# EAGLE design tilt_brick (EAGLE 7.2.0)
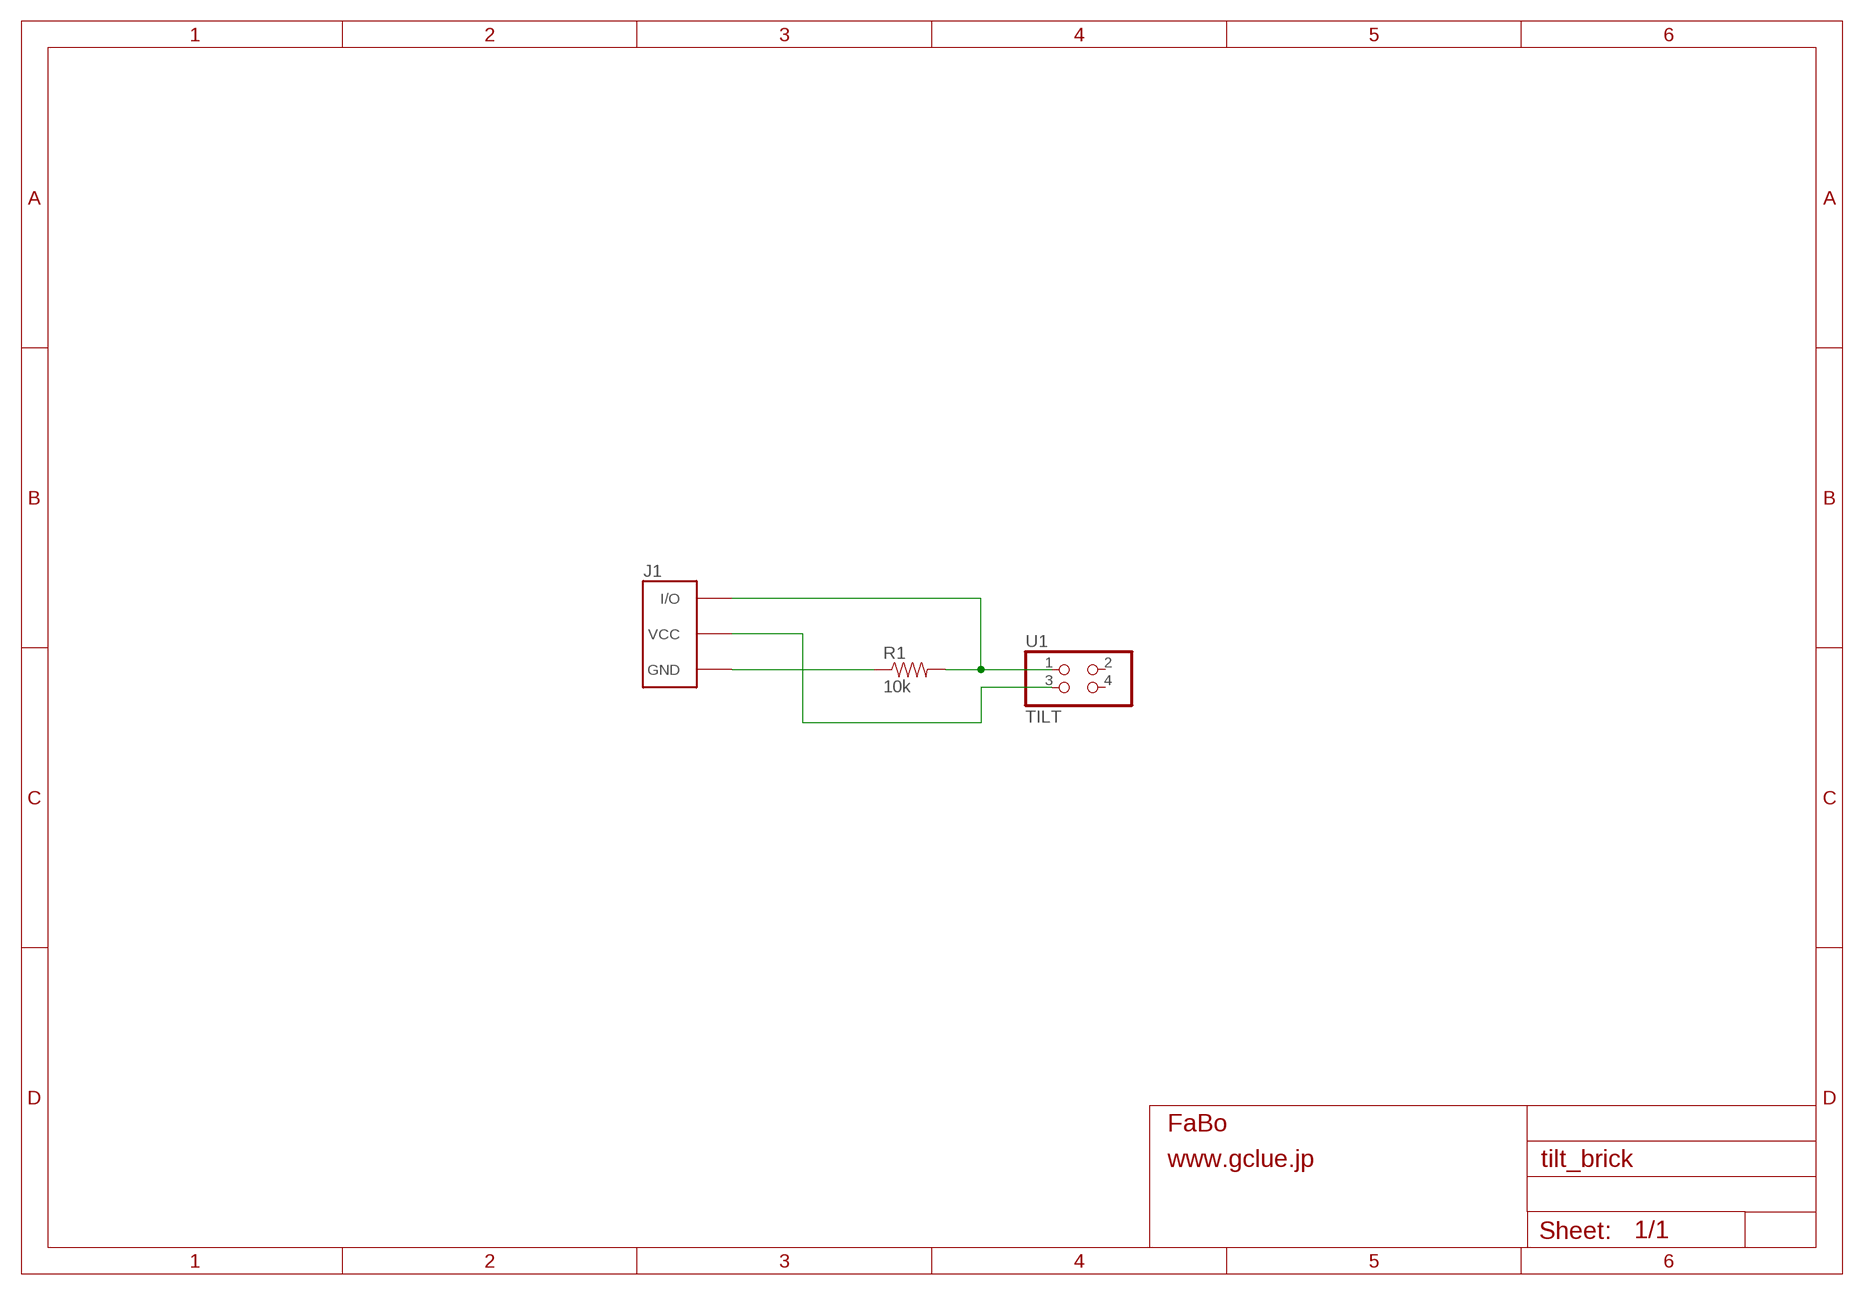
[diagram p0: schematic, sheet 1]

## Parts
J1  BRICK_3PIN  [BRICK_3PIN]
R1  10k  RESISTORKIT  [AXIAL-0.3-KIT]
U1  TILT  PINHD-2X2  [2X02]

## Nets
GND: J1.GND R1.P$1
N$3: J1.IN/OUT(I/O) R1.P$2 U1.1
N$5: J1.VCC U1.3
Unconnected: U1.2 U1.4

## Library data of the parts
J1 = Gclue:BRICK_3PIN: FaBo Brick 3pin
R1 = SparkFun:RESISTOR: Resistor
U1 = pinhead:PINHD-2X2: PIN HEADER

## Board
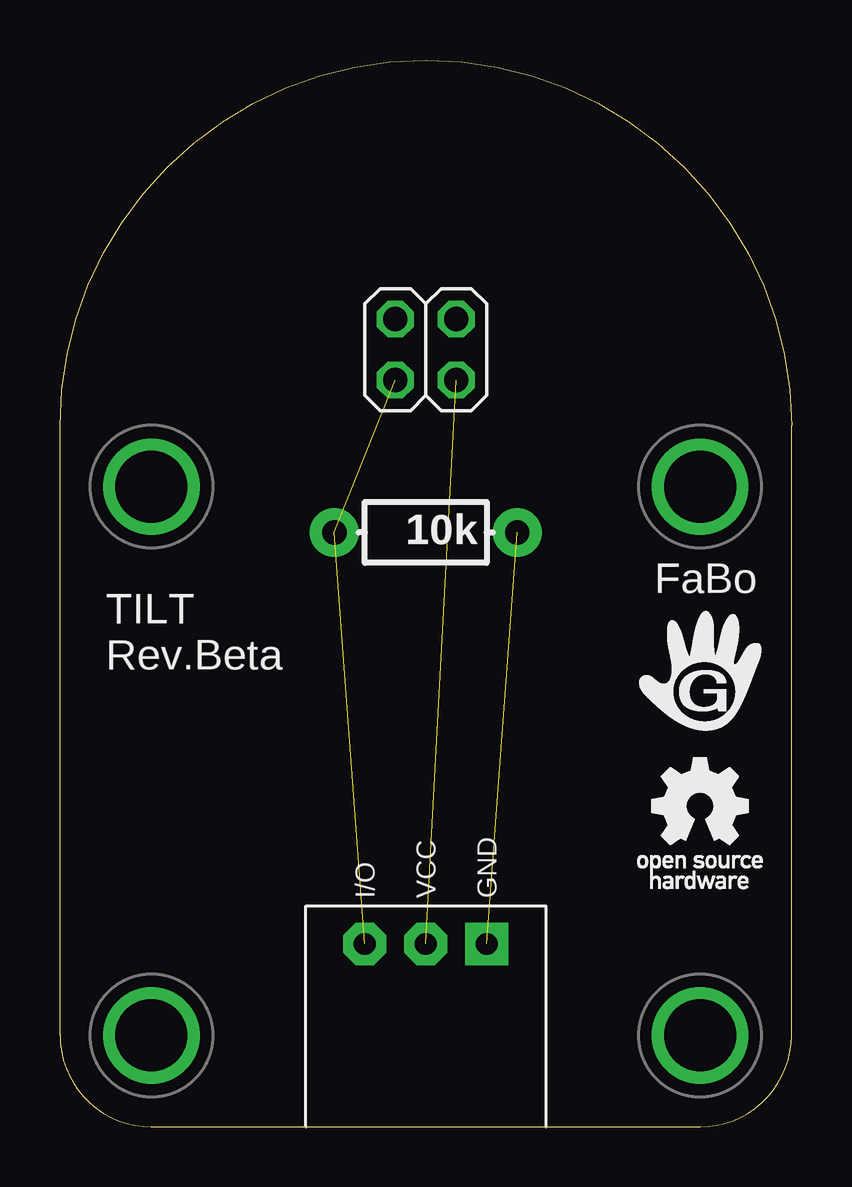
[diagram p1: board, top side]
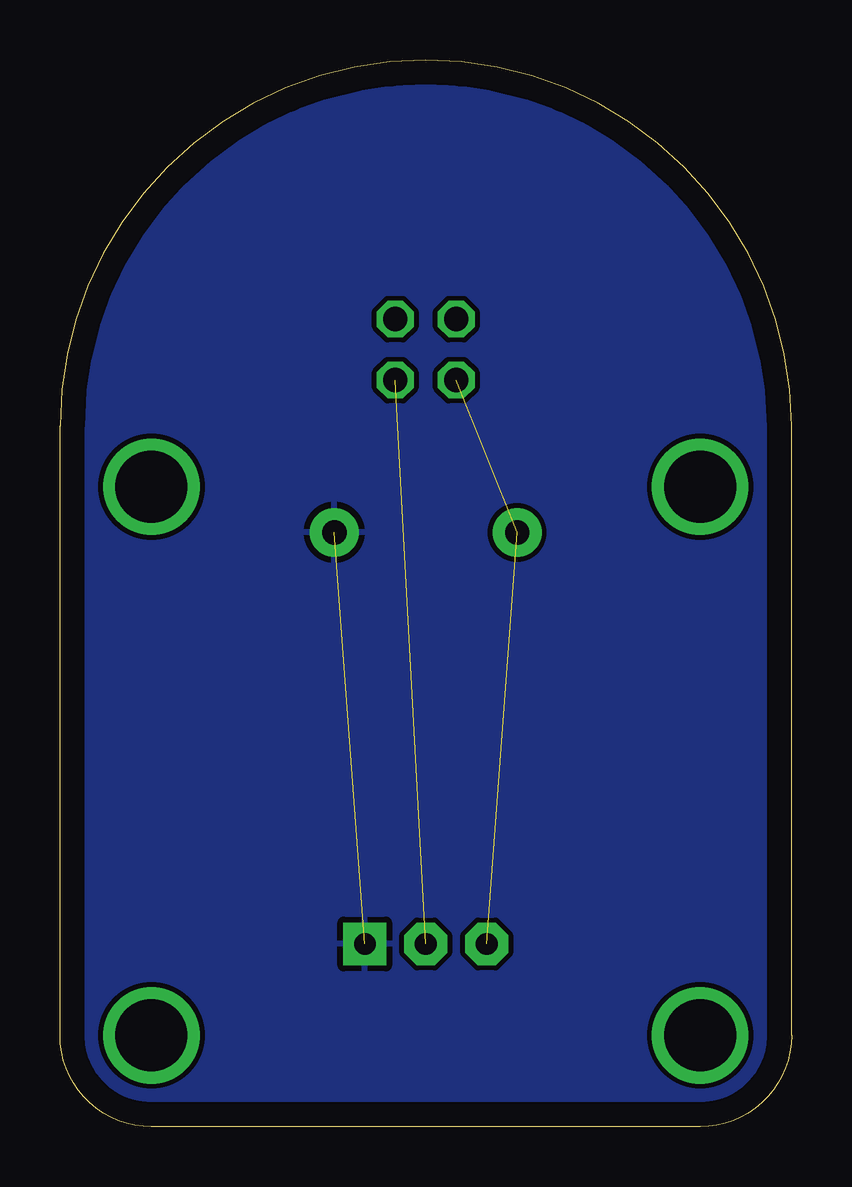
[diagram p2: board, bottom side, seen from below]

Size 30.48 x 44.45 mm. Coordinates in mm from the lower left corner, seen from the top.
Copper layers (1*16): Top 0.035mm / dielectric 1.5mm / Bottom 0.035mm
Design rules "default": minimum track width 10mil, minimum drill 24mil, track to track 8mil, track to pad 8mil, pad to pad 8mil, via to via 8mil, smd to smd 8mil, copper to edge 40mil, drill to drill 8mil, minimum pad ring 10mil, minimum via ring 8mil, stop-mask expansion 4mil, vias tented up to drill 0mil, thermal gap 10mil

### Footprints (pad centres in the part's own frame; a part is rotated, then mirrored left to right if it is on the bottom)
BRICK_3PIN = drill 0.9 pad 1.778 square: GND 2.54,-11.43 | drill 0.9 pad 1.778 octagon: IN/OUT -2.54,-11.43; VCC 0,-11.43 | drill 3 pad 3.81: P$1 -11.43,7.62; P$2 11.43,7.62; P$3 11.43,-15.24; P$4 -11.43,-15.24
AXIAL-0.3-KIT = drill 1.016 pad 2.032: P$1 -3.81,0; P$2 3.81,0
2X02 = drill 1.016 octagon: 1 -1.27,-1.27; 2 -1.27,1.27; 3 1.27,-1.27; 4 1.27,1.27

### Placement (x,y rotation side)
J1  15.24,19.05 0 top
R1  15.24,24.77 180 top
U1  15.24,32.38 0 top
U$2  [LOGO_OSHW_T_M]  26.67,13.34 0 top
U$3  [LOGO_GCLUE_M]  26.67,19.05 0 top

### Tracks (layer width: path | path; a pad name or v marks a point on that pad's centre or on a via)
GND  (1 unrouted)
  pour Bottom: 0,0 30.48,0 29.84,43.81 -0.64,44.45
N$3  (2 unrouted)
N$5  (1 unrouted)

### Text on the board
tPlace: FaBo | TILT / Rev.Beta

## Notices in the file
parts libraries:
SparkFun: Licensing: CC v3.0 Share-Alike You are welcome to use this library for commercial purposes.
